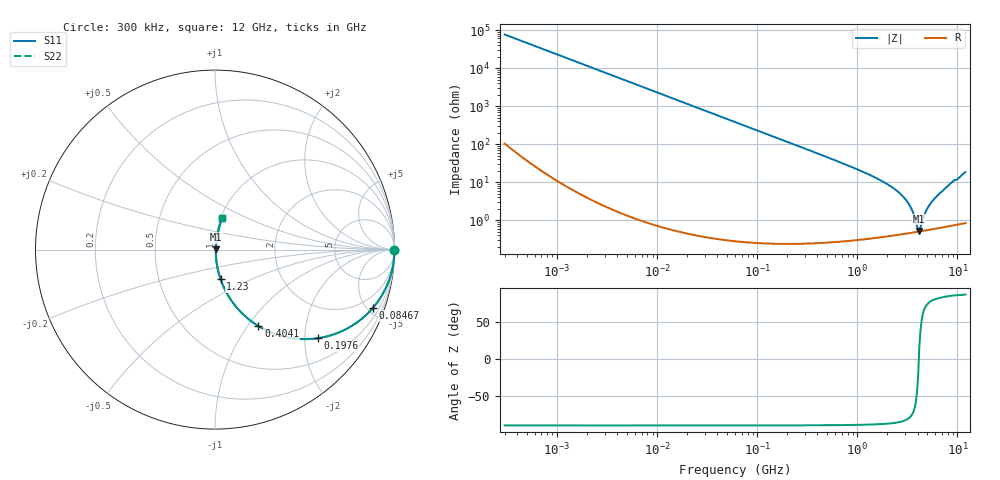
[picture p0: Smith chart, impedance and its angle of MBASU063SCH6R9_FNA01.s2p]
! MBASU063SCH6R9_FNA01  S-PARAMETER MODEL  ( General Type )
! Model Generated by TAIYO YUDEN Corporation (http://www.ty-top.com)
! Version 1.0
! TAIYO YUDEN Control No. 130801
! Copyright(c) 2013 TAIYO YUDEN CO.,LTD. All Rights Reserved.
! Product Description (link to TY-COMPAS)
! https://ds.yuden.co.jp/TYCOMPAS/or/detail?pn=MBASU063SCH6R9DFNA01&u=M
! Products Name : Multilayer Ceramic Capacitors
! Characteristics :
!  Capacitance : 6.9 pF , Rated Voltage : 50V , TCC : CH / C0H
!  Case Size : 0.6 x 0.3 / 0.024 x 0.012 [mm/inch] , Thickness : 0.3 / 0.012 [mm/inch]
!  (Conditions: Temperature = 25 degC , DC Bias Current/Voltage = 0A / 0V)
! External Node Assignments :
!  1  o---| |---o  2
! GND o---------o GND
! Frequency Range : 0.3MHz  -  12000MHz  [ 401 STEP ]
# MHz S RI R 50
! Freq[MHz].  S11 Real  S11 Imag  S21 Real  S21 Imag  S12 Real  S12 Imag  S22 Real  S22 Imag
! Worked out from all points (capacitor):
!   401 points, 300 kHz to 12 GHz, reference 50 ohm
!   read as one part in series: C = 6.93 pF near 316.3 kHz
!   lowest |Z| = 523 mohm at 4.159 GHz (marker M1)
!   series resonance near 4.114 GHz, so ESL is about 220 pH
!   S11 on the Smith chart (normalised r, x): 300 kHz: open; 84.67 MHz: 1.01, -5.42; 197.6 MHz: 1.00, -2.32; 404.1 MHz: 1.00, -1.13; 1.23 GHz: 1.01, -0.34; 12 GHz: 1.02, +0.37
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0.3  1 -0.00131  3.47e-06 0.00131  3.47e-06 0.00131  1 -0.00131
1.769972  0.9999 -0.00771  6.21e-05 0.00771  6.21e-05 0.00771  0.9999 -0.00771
10.44266  0.9979 -0.0454  0.00208 0.0454  0.00208 0.0454  0.9979 -0.0454
27.10171  0.9862 -0.1164  0.0138 0.1164  0.0138 0.1164  0.9862 -0.1164
60  0.9359 -0.2446  0.0641 0.2446  0.0641 0.2446  0.9359 -0.2446
84.66778  0.88 -0.3245  0.12 0.3245  0.12 0.3245  0.88 -0.3245
197.6437  0.5731 -0.4936  0.4269 0.4936  0.4269 0.4936  0.5731 -0.4936
353.9943  0.2938 -0.4536  0.7062 0.4536  0.7062 0.4536  0.2938 -0.4536
404.1309  0.2415 -0.4258  0.7585 0.4258  0.7585 0.4258  0.2415 -0.4258
668.5285  0.1025 -0.2993  0.8975 0.2993  0.8975 0.2993  0.1025 -0.2993
1229.528  0.031 -0.1643  0.969 0.1643  0.969 0.1643  0.031 -0.1643
2088.533  0.0103 -0.0806  0.9897 0.0806  0.9897 0.0806  0.0103 -0.0806
2650.866  0.00669 -0.0503  0.9933 0.0503  0.9933 0.0503  0.00669 -0.0503
3107.553  0.00542 -0.0316  0.9946 0.0316  0.9946 0.0316  0.00542 -0.0316
3547.679  0.00495 -0.0166  0.9951 0.0166  0.9951 0.0166  0.00495 -0.0166
3944.255  0.00491 -0.00489  0.9951 0.00489  0.9951 0.00489  0.00491 -0.00489
4158.869  0.005 0.00143  0.995 -0.00143  0.995 -0.00143  0.005 0.00143
4270.516  0.00507 0.004  0.9949 -0.004  0.9949 -0.004  0.00507 0.004
4875.354  0.00565 0.0168  0.9944 -0.0168  0.9944 -0.0168  0.00565 0.0168
5715.274  0.00683 0.0325  0.9932 -0.0325  0.9932 -0.0325  0.00683 0.0325
8732.115  0.0163 0.0951  0.9837 -0.0951  0.9837 -0.0951  0.0163 0.0951
12000  0.0403 0.1752  0.9597 -0.1752  0.9597 -0.1752  0.0403 0.1752
